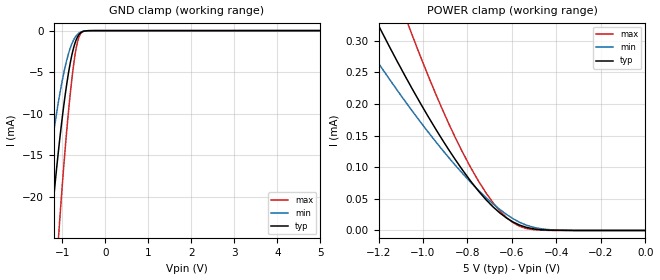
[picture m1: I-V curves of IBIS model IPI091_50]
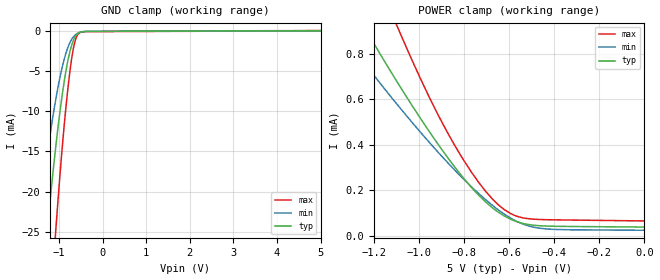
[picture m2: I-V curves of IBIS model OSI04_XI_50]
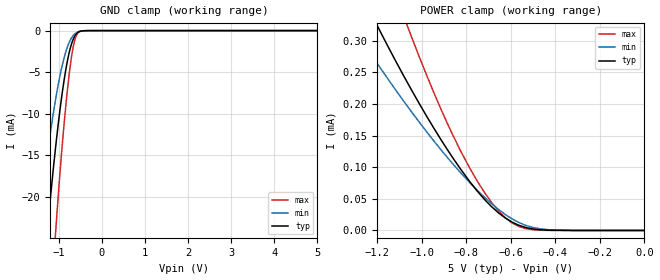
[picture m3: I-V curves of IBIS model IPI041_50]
| TEXAS INSTRUMENTS INCORPORATED
| Connectivity Solutions Group
| IBIS Model of TL16C550DRHB_5V
| 550D_RHB_5V
| This file contains package information for the following:
|  RHB 32-pin (QFN) package as [Component] 550DRHB_5V
| This device can be powered at the following Vccs:
|  5.0 Volt Vcc
| This file provides unique models under the [Model Selector] for each Vcc.
| For operation at a specific Vcc, select the appropriate model after each
| [Model Selector] keyword.
[IBIS Ver]   3.2
[Comment char]  |_char
[File Name]   550D_RHB_5V.ibs
[File Rev]   1 | a
[Date]   January 5, 2009
[Source]   Data created from TI-SPICE simulations at TI-CONN.
[Notes]   The following is an IBIS list for the 550D_RHB_5V.
   Please contact s-ly@ti.com with questions and
   comments concerning CONN IBIS models.
[Disclaimer] Property of Texas Instruments Incorporated.  Unauthorized
   reproduction and/or distribution is strictly prohibited.
   This product is protected under copyright law.
   Created  2003, (C) Copyright  2003, Texas Instruments
   Incorporated, All Rights Reserved
   UNLESS THERE IS A SIGNED, WRITTEN AGREEMENT TO THE
   CONTRARY, TEXAS INSTRUMENTS (TI) IS PROVIDING THE IBIS
   MODELS  AND WITHOUT ANY WARRANTY, EXPRESSED OR
   IMPLIED.  TI assumes no liability for:
   1) the accuracy of the IBIS models provided to your
   company;
   2) the proper functioning of these IBIS Models in your
   design or for any resulting applications; or
   3) infringement of patents, copyrights or intellectual
   property rights resulting from your use of these IBIS
   models.
   TI provides IBIS Models as a service to our customers.
   You and your company shall not distribute, sell or give
   these models to anyone else without prior written
   permission from TI.
   TI reserves the right to make changes to our products or
   to discontinue any semiconductor product or service
   without notice, and advises our customers to obtain the
   latest version of relevant information to verify, before
   placing orders, that the information being relied on is
   current.
   Please be aware that your receipt and use of the IBIS
   information provided shall serve as acceptance of these
   terms and conditions.  If you do not accept these terms,
   you should return or destroy the IBIS models and any
   other accompanying information immediately.
| Component 550D_5V_RHB 32-pin QFN
[Component]   550D_RHB_5V
[Manufacturer]   Texas Instruments, Inc.
[Package]
|   typ   min   max
R_pkg   4.900e-04   4.900e-04   4.900e-04
L_pkg   1.009e-10   0.683e-10   1.336e-10
C_pkg   2.424e-14   1.463e-14   3.850e-14
[Pin]   signal_name   model_name   R_pin   L_pin   C_pin
1   D4   IPI04_OPJ43   4.900e-04   1.347e-10   8.118e-14
2   NC   NC   4.900e-04   1.284e-10   9.657e-14
3   D5   IPI04_OPJ43   4.900e-04   1.275e-10   9.662e-14
4   D6   IPI04_OPJ43   4.900e-04   1.273e-10   9.663e-14
5   D7   IPI04_OPJ43   4.900e-04   1.273e-10   9.663e-14
6   SIN   IPI041   4.900e-04   1.275e-10   9.661e-14
7   SOUT   OPJ430   4.900e-04   1.285e-10   9.656e-14
8   CS2B   IPI041   4.900e-04   1.347e-10   8.119e-14
9   NC   NC   4.900e-04   1.347e-10   8.118e-14
10   XIN   OSI04_XI   4.900e-04   1.284e-10   9.657e-14
11   XOUT   OSI04   4.900e-04   1.275e-10   9.662e-14
12   WR1B   IPI041   4.900e-04   1.273e-10   9.663e-14
13   VSS   GND   4.900e-04   1.273e-10   9.663e-14
14   RD1B   IPI041   4.900e-04   1.275e-10   9.660e-14
15   NC   NC   4.900e-04   1.285e-10   9.653e-14
16   NC   NC   4.900e-04   1.348e-10   8.116e-14
17   A2   IPI041   4.900e-04   1.348e-10   8.117e-14
18   A1   IPI041   4.900e-04   1.285e-10   9.656e-14
19   A0   IPI041   4.900e-04   1.275e-10   9.661e-14
20   INTRPT   OPJ430   4.900e-04   1.273e-10   9.662e-14
21   RTSB   OPJ430   4.900e-04   1.273e-10   9.662e-14
22   DTRB   OPJ430   4.900e-04   1.275e-10   9.663e-14
23   MR   IPI091   4.900e-04   1.284e-10   9.657e-14
24   CTSB   IPI041   4.900e-04   1.347e-10   8.117e-14
25   DSRB   IPI041   4.900e-04   1.348e-10   8.117e-14
26   DCDB   IPI041   4.900e-04   1.285e-10   9.656e-14
27   RIB   IPI041   4.900e-04   1.275e-10   9.662e-14
28   VCC   POWER   4.900e-04   1.273e-10   9.663e-14
29   D0   IPI04_OPJ43   4.900e-04   1.273e-10   9.662e-14
30   D1   IPI04_OPJ43   4.900e-04   1.275e-10   9.663e-14
31   D2   IPI04_OPJ43   4.900e-04   1.284e-10   9.657e-14
32   D3   IPI04_OPJ43   4.900e-04   1.348e-10   8.116e-14
| Model IPI091
[Model Selector]   IPI091
IPI091_50   5 volt Vcc
| Model OSI04_XI
[Model Selector]   OSI04_XI
OSI04_XI_50   5 volt Vcc
| Model IPI041
[Model Selector]   IPI041
IPI041_50   5 volt Vcc
| Model IPI04_OPJ43
[Model Selector]   IPI04_OPJ43
IPI04_OPJ43_50   5 volt Vcc
| Model OPJ430
[Model Selector]   OPJ430
OPJ430_50   5 volt Vcc
| Model OSI04
[Model Selector]   OSI04
OSI04_50   5 volt Vcc
| Models and submodels in the file (6): IPI091_50 (Input), OSI04_XI_50 (Input), IPI041_50 (Input), IPI04_OPJ43_50 (I/O), OPJ430_50 (3-state), OSI04_50 (3-state)
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[Model]   IPI091_50
Model_type  Input
Vinl = 0
Vinh = 5
| variable   typ   min   max
C_comp   1.05pF   0.91pF   1.20pF
[Temperature Range]   40   125   -40
| Ambient temperature   25   110   -40
[Voltage range]   5   4.5   5.5
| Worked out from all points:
|   GND clamp passes 1 mA (typ) near -0.66 V on its own axis
|   POWER clamp passes 1 mA (typ) near -2.02 V on its own axis
[GND Clamp]
| IPI091_50
|   Voltage   I(typ)   I(min)   I(max)
-5V       -337.5mA   -249.9mA   -446.9mA
-1.485V   -37.43mA   -23.94mA   -59.12mA
-1.27V    -24.21mA   -14.96mA   -39.8mA
-1.085V   -14.44mA   -8.531mA   -24.93mA
-1.065V   -13.5mA    -7.923mA   -23.45mA
-920mV    -7.399mA   -4.126mA   -13.63mA
-845mV    -4.864mA   -2.644mA   -9.318mA
-775mV    -2.962mA   -1.595mA   -5.878mA
-665mV    -1.007mA   -578.3uA   -1.875mA
-570mV    -262.1uA   -185.2uA   -368.6uA
-400mV    -8.531uA   -12.92uA   -6.748uA
5V        489.4pA    4.684uA    103.1pA
[POWER Clamp]
| IPI091_50
|   Voltage   I(typ)   I(min)   I(max)
-5V       7.166mA    6.06mA     10.13mA
-1.305V   398.7uA    319.9uA    565.1uA
-1.185V   313.6uA    256.4uA    440.3uA
-1.08V    243.8uA    203.9uA    337.8uA
-1.045V   221.6uA    187.1uA    305.3uA
-915mV    144.4uA    128.2uA    193uA
-785mV    77.58uA    75.9uA     99.02uA
-715mV    47.95uA    51.41uA    58.45uA
-625mV    19.85uA    25.4uA     20.38uA
-565mV    8.395uA    12.83uA    6.553uA
-465mV    1.046uA    2.445uA    370.2nA
-84.4fV   489.4pA    3.799nA    117.2pA
[Model]   OSI04_XI_50
Model_type  Input
Vinl = 0
Vinh = 5
| variable   typ   min   max
C_comp   1.87pF   1.18pF   2.42pF
[Temperature Range]   40   125   -40
| Ambient temperature   25   110   -40
[Voltage range]   5   4.5   5.5
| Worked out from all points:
|   GND clamp passes 1 mA (typ) near -0.66 V on its own axis
|   POWER clamp passes 1 mA (typ) near -1.29 V on its own axis
[GND Clamp]
| OSI04_XI_50
|   Voltage   I(typ)   I(min)   I(max)
-5V       -343.1mA   -253.2mA   -455.7mA
-1.525V   -41.07mA   -26.37mA   -64.46mA
-1.48V    -38.05mA   -24.29mA   -60.12mA
-1.265V   -24.63mA   -15.21mA   -40.45mA
-1.085V   -14.94mA   -8.861mA   -25.7mA
-1.065V   -13.97mA   -8.241mA   -24.18mA
-915mV    -7.534mA   -4.251mA   -13.83mA
-770mV    -3.03mA    -1.696mA   -5.942mA
-665mV    -1.111mA   -697uA     -2.029mA
-565mV    -298uA     -251.7uA   -421.3uA
-390mV    -48.3uA    -40.46uA   -75.23uA
5V        38.17uA    39.29uA    59.24uA
[POWER Clamp]
| OSI04_XI_50
|   Voltage   I(typ)   I(min)   I(max)
-5V       11.35mA    8.695mA    16.41mA
-1.365V   1.132mA    919.8uA    1.585mA
-1.25V    930.2uA    769uA      1.291mA
-1.215V   870.6uA    724.2uA    1.204mA
-1.115V   705.4uA    599.5uA    963.5uA
-1.085V   657.4uA    563.1uA    893.9uA
-945mV    444.6uA    400.2uA    590.1uA
-800mV    250.3uA    246.8uA    329.3uA
-705mV    148.8uA    158.9uA    196uA
-620mV    86.09uA    93.87uA    113.7uA
-465mV    43.98uA    32.94uA    71.4uA
-84.4fV   38.17uA    24.06uA    65.18uA
[Model]   IPI041_50
Model_type  Input
Vinl = 0
Vinh = 5
| variable   typ   min   max
C_comp   1.06pF   0.91pF   1.20pF
[Temperature Range]   40   125   -40
| Ambient temperature   25   110   -40
[Voltage range]   5   4.5   5.5
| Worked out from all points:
|   GND clamp passes 1 mA (typ) near -0.66 V on its own axis
|   POWER clamp passes 1 mA (typ) near -2.02 V on its own axis
[GND Clamp]
| IPI041_50
|   Voltage   I(typ)   I(min)   I(max)
-5V       -337.5mA   -249.9mA   -446.9mA
-1.485V   -37.43mA   -23.94mA   -59.12mA
-1.27V    -24.21mA   -14.96mA   -39.8mA
-1.085V   -14.44mA   -8.531mA   -24.93mA
-1.065V   -13.5mA    -7.923mA   -23.45mA
-920mV    -7.399mA   -4.126mA   -13.63mA
-845mV    -4.864mA   -2.644mA   -9.318mA
-775mV    -2.962mA   -1.595mA   -5.878mA
-665mV    -1.007mA   -578.3uA   -1.875mA
-570mV    -262.1uA   -185.2uA   -368.6uA
-400mV    -8.531uA   -12.92uA   -6.748uA
5V        489.4pA    4.684uA    103.1pA
[POWER Clamp]
| IPI041_50
|   Voltage   I(typ)   I(min)   I(max)
-5V       7.166mA    6.06mA     10.13mA
-1.305V   398.7uA    319.9uA    565.1uA
-1.185V   313.6uA    256.4uA    440.3uA
-1.08V    243.8uA    203.9uA    337.8uA
-1.045V   221.6uA    187.1uA    305.3uA
-915mV    144.4uA    128.2uA    193uA
-785mV    77.58uA    75.9uA     99.02uA
-715mV    47.95uA    51.41uA    58.45uA
-625mV    19.85uA    25.4uA     20.38uA
-565mV    8.395uA    12.83uA    6.553uA
-465mV    1.046uA    2.445uA    370.2nA
-84.4fV   489.4pA    3.799nA    117.2pA
